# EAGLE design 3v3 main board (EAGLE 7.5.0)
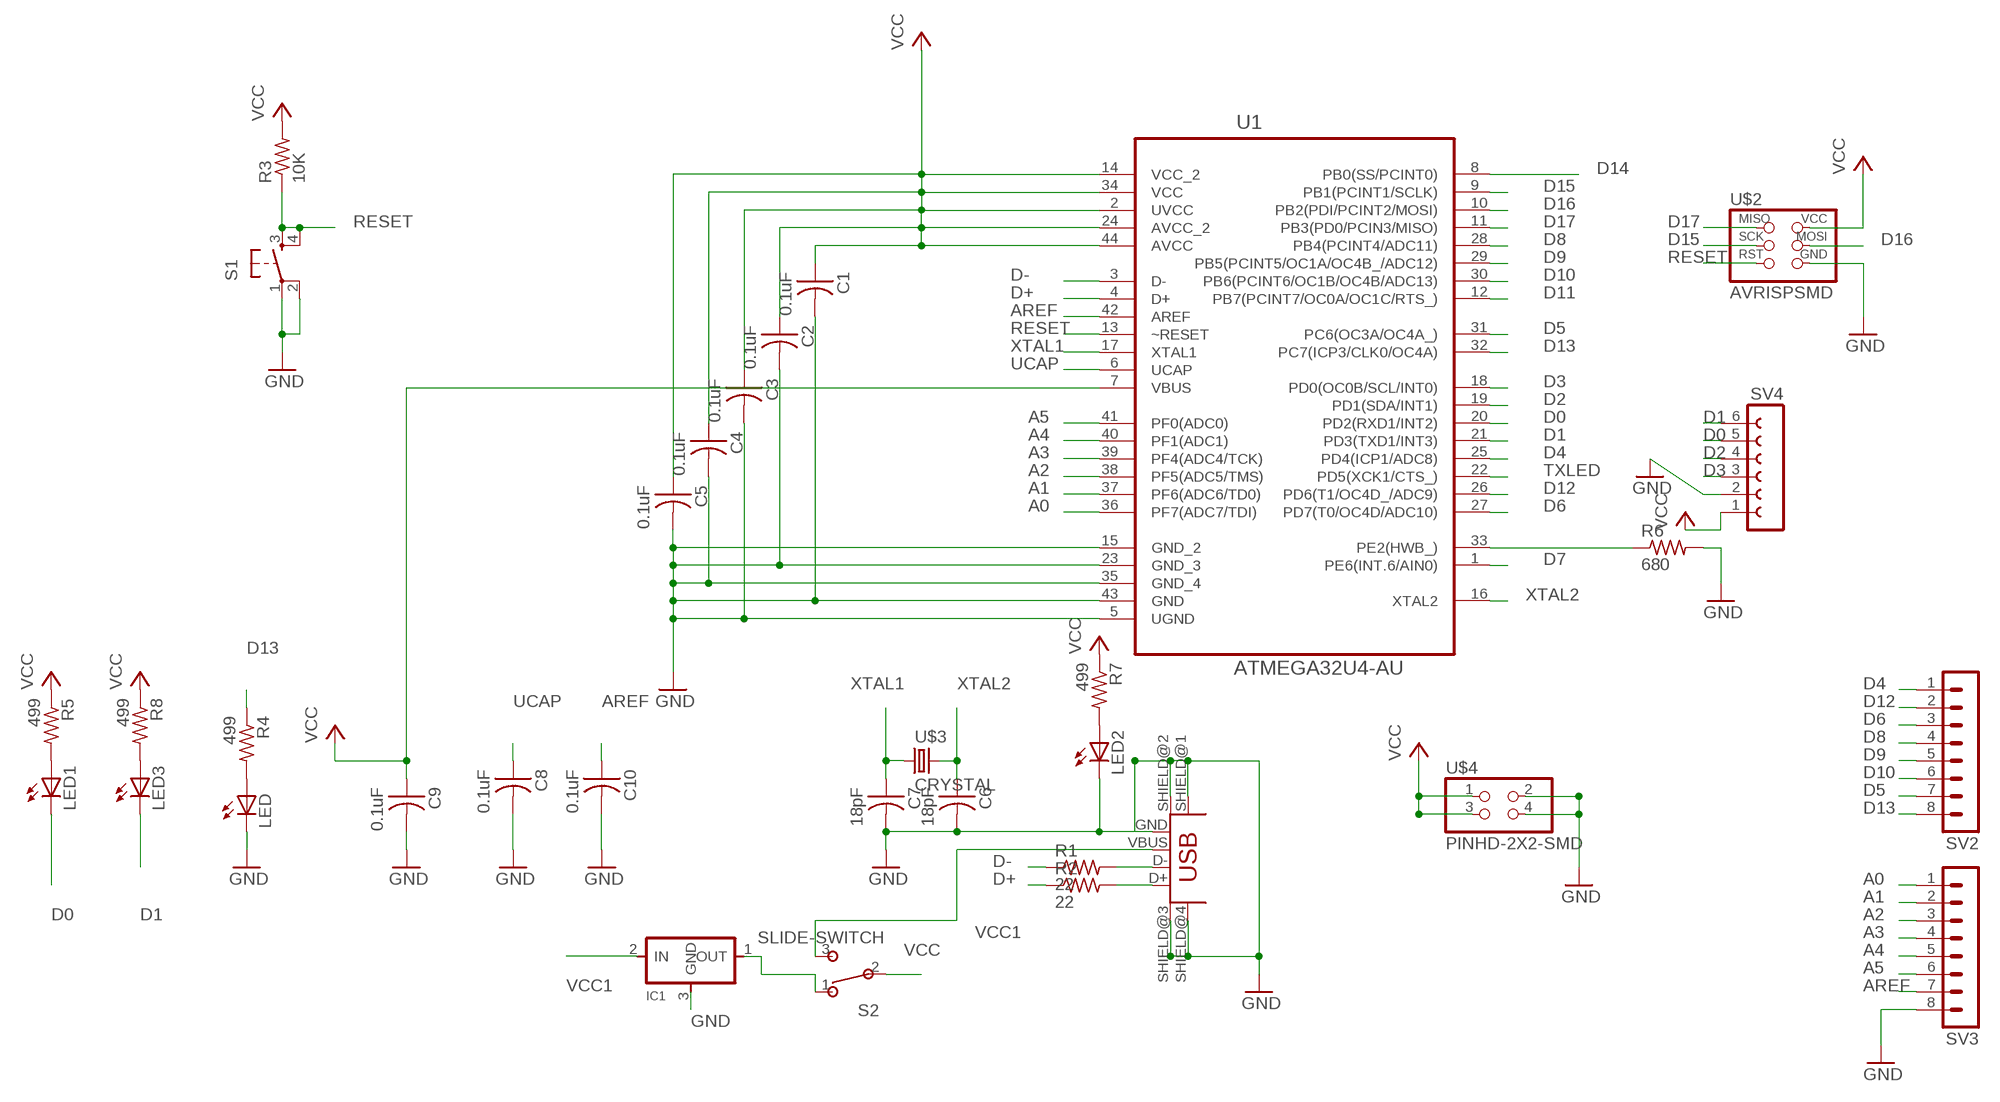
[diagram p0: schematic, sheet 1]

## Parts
C1  0.1uF  CAP-US1206FAB  [C1206FAB]
C2  0.1uF  CAP-US1206FAB  [C1206FAB]
C3  0.1uF  CAP-US1206FAB  [C1206FAB]
C4  0.1uF  CAP-US1206FAB  [C1206FAB]
C5  0.1uF  CAP-US1206FAB  [C1206FAB]
C6  18pF  CAP-US1206FAB  [C1206FAB]
C7  18pF  CAP-US1206FAB  [C1206FAB]
C8  0.1uF  CAP-US1206FAB  [C1206FAB]
C9  0.1uF  CAP-US1206FAB  [C1206FAB]
C10  0.1uF  CAP-US1206FAB  [C1206FAB]
IC1  REGULATORSOT23  [SOT23]
LED  LED1206  [1206]
LED1  LED1206  [1206]
LED2  LED1206  [1206]
LED3  LED1206  [1206]
R1  22  RES-US1206FAB  [R1206FAB]
R2  22  RES-US1206FAB  [R1206FAB]
R3  10K  RES-US1206FAB  [R1206FAB]
R4  499  RESISTOR1206  [1206]
R5  499  RESISTOR1206  [1206]
R6  680  RES-US1206FAB  [R1206FAB]
R7  499  RESISTOR1206  [1206]
R8  499  RESISTOR1206  [1206]
S1  6MM_SWITCH6MM_SWITCH  [6MM_SWITCH]
S2  SLIDE-SWITCH  [AYZ0102AGRLC]
SV2  MA08-1  [MA08-1]
SV3  MA08-1  [MA08-1]
SV4  FE06-1  [FE06]
U1  ATMEGA32U4-AU  [QFP80P1200X1200X120-44N]
U$1  USB_MINIB  [USB_MINIB]
U$2  AVRISPSMD  [2X03SMD]
U$3  CRYSTAL  [2-SMD-5X3MM]
U$4  PINHD-2X2-SMD  [2X02SMD]

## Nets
A0: SV3.1 U1.36(PF7(ADC7/TDI))
A1: SV3.2 U1.37(PF6(ADC6/TD0))
A2: SV3.3 U1.38(PF5(ADC5/TMS))
A3: SV3.4 U1.39(PF4(ADC4/TCK))
A4: SV3.5 U1.40(PF1(ADC1))
A5: SV3.6 U1.41(PF0(ADC0))
AREF: C10.1 SV3.7 U1.42(AREF)
D0: LED1.2(C) SV4.5 U1.20(PD2(RXD1/INT2))
D1: LED3.2(C) SV4.6 U1.21(PD3(TXD1/INT3))
D2: SV4.4 U1.19(PD1(SDA/INT1))
D3: SV4.3 U1.18(PD0(OC0B/SCL/INT0))
D4: SV2.1 U1.25(PD4(ICP1/ADC8))
D5: SV2.7 U1.31(PC6(OC3A/OC4A_))
D6: SV2.3 U1.27(PD7(T0/OC4D/ADC10))
D7: U1.1(PE6(INT.6/AIN0))
D8: SV2.4 U1.28(PB4(PCINT4/ADC11))
D9: SV2.5 U1.29(PB5(PCINT5/OC1A/OC4B_/ADC12))
D10: SV2.6 U1.30(PB6(PCINT6/OC1B/OC4B/ADC13))
D11: U1.12(PB7(PCINT7/OC0A/OC1C/RTS_))
D12: SV2.2 U1.26(PD6(T1/OC4D_/ADC9))
D13: R4.1 SV2.8 U1.32(PC7(ICP3/CLK0/OC4A))
D14: U1.8(PB0(SS/PCINT0))
D15: U1.9(PB1(PCINT1/SCLK)) U$2.3(SCK)
D16: U1.10(PB2(PDI/PCINT2/MOSI)) U$2.4(MOSI)
D17: U1.11(PB3(PD0/PCIN3/MISO)) U$2.1(MISO)
D+: R2.1 U1.4(D+)
D-: R1.1 U1.3(D-)
GND: C1.2 C2.2 C3.2 C4.2 C5.2 C6.2 C7.2 C8.2 C9.2 C10.2 IC1.3(GND) LED2.2(C) LED.2(C) R6.2 S1.1(P) S1.2(P1) SV3.8 SV4.2 U1.5(UGND) U1.15(GND_2) U1.23(GND_3) U1.35(GND_4) U1.43(GND) U$1.GND U$1.SHIELD@1(SHIELD) U$1.SHIELD@2(SHIELD1) U$1.SHIELD@3(SHIELD2) U$1.SHIELD@4(SHIELD3) U$2.6(GND) U$4.2 U$4.4
N$1: R1.2 U$1.D-
N$2: R2.2 U$1.D+
N$3: LED.1(A) R4.2
N$4: LED1.1(A) R5.2
N$5: LED2.1(A) R7.2
N$6: LED3.1(A) R8.2
N$10: IC1.1(OUT) S2.1
N$35: R6.1 U1.33(PE2(HWB_))
RESET: R3.1 S1.3(S) S1.4(S1) U1.13(~RESET) U$2.5(RST)
TXLED: U1.22(PD5(XCK1/CTS_))
UCAP: C8.1 U1.6(UCAP)
VCC: C1.1 C2.1 C3.1 C4.1 C5.1 C9.1 R3.2 R5.1 R7.1 R8.1 S2.2 SV4.1 U1.2(UVCC) U1.7(VBUS) U1.14(VCC_2) U1.24(AVCC_2) U1.34(VCC) U1.44(AVCC) U$2.2(VCC) U$4.1 U$4.3
VCC1: IC1.2(IN) S2.3 U$1.VBUS
XTAL1: C7.1 U1.17(XTAL1) U$3.P$1
XTAL2: C6.1 U1.16(XTAL2) U$3.P$2

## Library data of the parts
C1-C10 = fab:CAP-US
IC1 = fab:REGULATOR
LED LED1-LED3 = ng:LED
R1-R3 R6 = fab:RES-US: Resistor (US Symbol)
R4 R5 R7 R8 = ng:RESISTOR
S1 = ng:6MM_SWITCH: OMRON SWITCH
S2 = fab:SLIDE-SWITCH: SMD slide-switch AYZ0102AGRLC as found in the fablab inventory. Includes the mounting holes. Made by Zaerc.
SV2 SV3 = con-lstb:MA08-1: PIN HEADER; OC_FARNELL: unknown; OC_NEWARK: unknown
SV4 = con-lsta:FE06-1: FEMALE HEADER; OC_FARNELL: unknown; OC_NEWARK: unknown
U1 = Atmel_By_element14_Batch_1:ATMEGA32U4-AU: 8-bit Microcontroller with ISP Flash and USB Controller; MPN: ATMEGA32U4-AU; OC_FARNELL: 1748525; OC_NEWARK: 26R5633; PACKAGE: TQFP-44; SUPPLIER: Atmel
U$1 = fab:USB_MINIB
U$2 = fab:AVRISP
U$3 = fab:CRYSTAL
U$4 = fab:PINHD-2X2-SMD

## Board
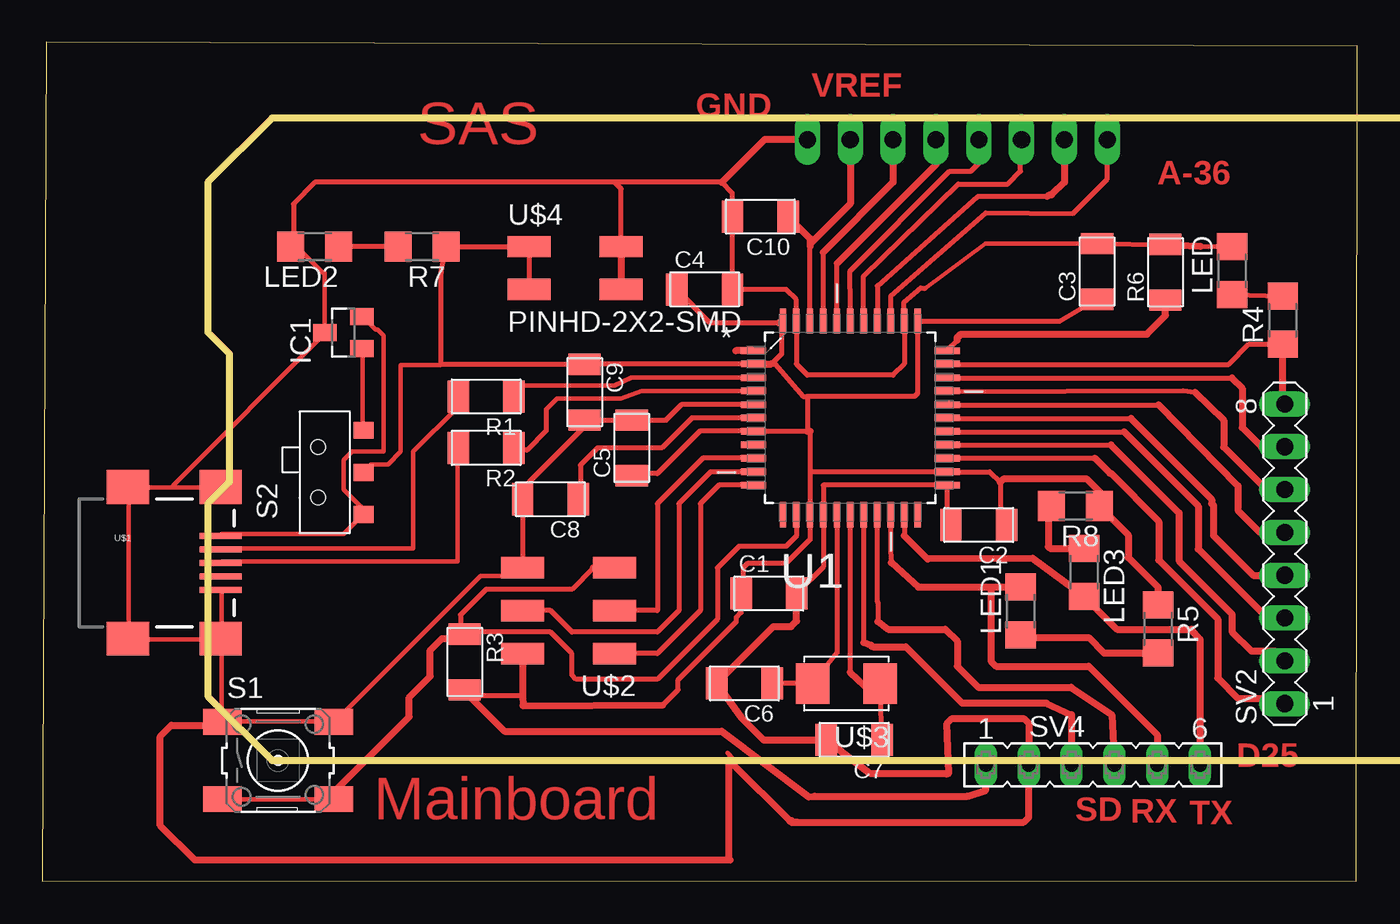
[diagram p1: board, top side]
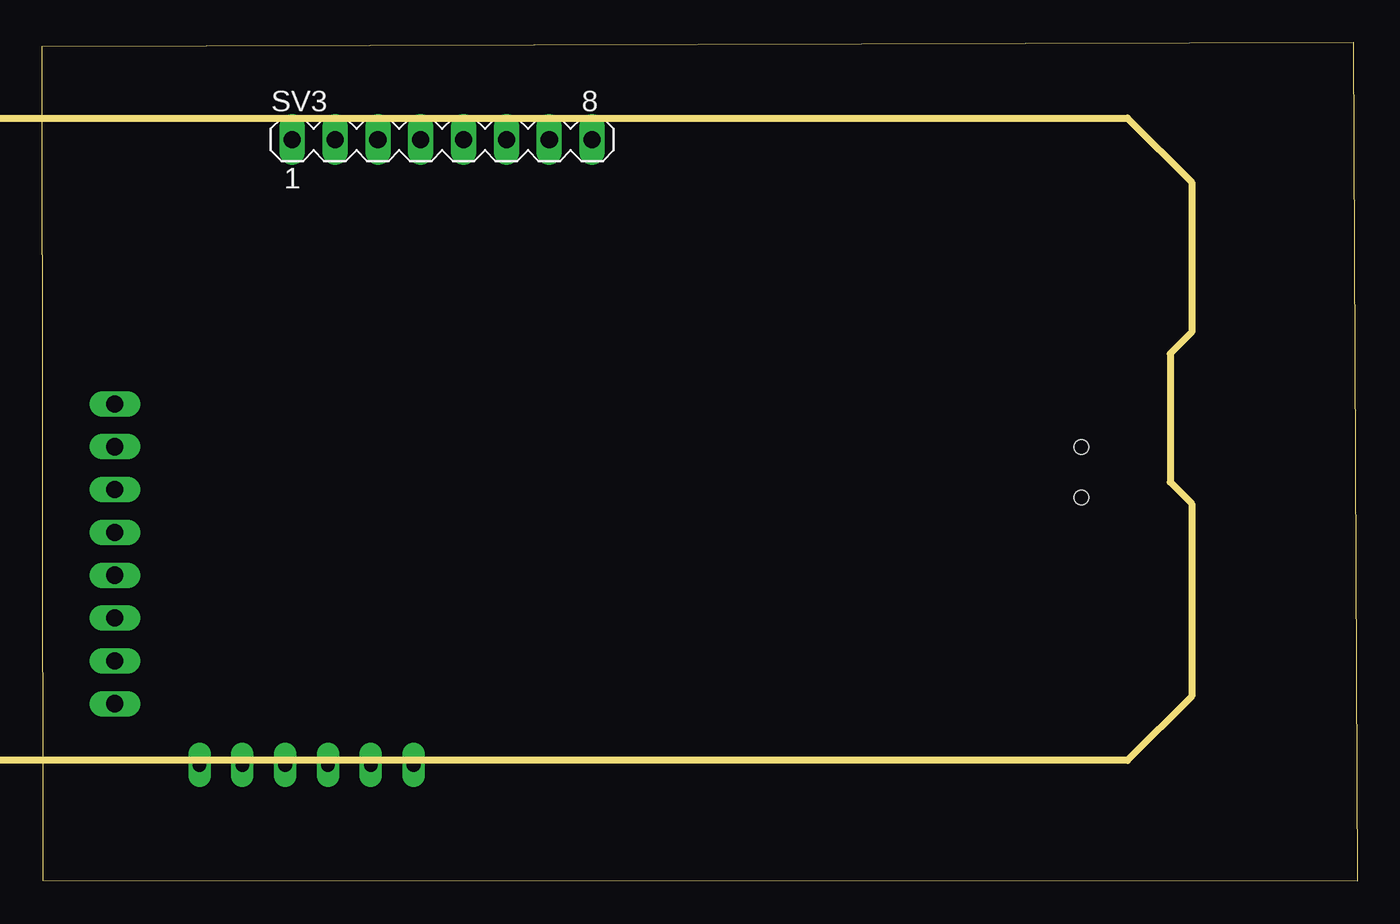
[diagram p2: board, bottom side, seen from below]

Size 77.99 x 49.78 mm. Coordinates in mm from the lower left corner, seen from the top.
Outline: 0,0 77.94,0.05 77.99,49.53 0.25,49.78 0,0
Copper layers (1*16): Top 0.035mm / dielectric 1.5mm / Bottom 0.035mm
Design rules "default *": minimum track width 10mil, minimum drill 24mil, track to track 0.4mm, track to pad 0.4mm, pad to pad 0.4mm, via to via 0.4mm, smd to smd 0.4mm, copper to edge 40mil, drill to drill 0.4mm, minimum pad ring 10mil, minimum via ring 8mil, stop-mask expansion 4mil, vias tented up to drill 0mil, thermal gap 10mil
Milling: area 9.8,7.2 to 110.2,45.3

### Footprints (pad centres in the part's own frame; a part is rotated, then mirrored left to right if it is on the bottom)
C1206FAB = smd 1.27 x 1.905: 1 -1.651,0; 2 1.651,0
SOT23 = smd 1 x 1.4: 1 -0.95,-1.1; 2 0.95,-1.1; 3 0,1.1
1206 = smd 1.6 x 1.803: 1 -1.422,0; 2 1.422,0
R1206FAB = smd 1.27 x 1.905: 1 -1.651,0; 2 1.651,0
6MM_SWITCH = smd 2.286 x 1.524: 1 -3.302,2.286; 2 3.302,2.286; 3 -3.302,-2.286; 4 3.302,-2.286
AYZ0102AGRLC = smd 1 x 1.2: 1 2.5,-2.3; 2 0,-2.3; 3 -2.5,-2.3 | hole 0.85: -1.5,0.4; 1.5,0.4
MA08-1 = drill 1.016 long: 1 -8.89,0; 2 -6.35,0; 3 -3.81,0; 4 -1.27,0; 5 1.27,0; 6 3.81,0; 7 6.35,0; 8 8.89,0
FE06 = drill 0.813 long: 1 -6.35,0; 2 -3.81,0; 3 -1.27,0; 4 1.27,0; 5 3.81,0; 6 6.35,0
QFP80P1200X1200X120-44N = smd 1.5 x 0.38: 1 -5.74,3.988; 2 -5.74,3.2; 3 -5.74,2.388; 4 -5.74,1.6; 5 -5.74,0.787; 6 -5.74,0; 7 -5.74,-0.787; 8 -5.74,-1.6; 9 -5.74,-2.388; 10 -5.74,-3.2; 11 -5.74,-3.988; 23 5.74,-3.988; 24 5.74,-3.2; 25 5.74,-2.388; 26 5.74,-1.6; 27 5.74,-0.787; 28 5.74,0; 29 5.74,0.787; 30 5.74,1.6; 31 5.74,2.388; 32 5.74,3.2; 33 5.74,3.988 | smd 0.38 x 1.5: 12 -3.988,-5.74; 13 -3.2,-5.74; 14 -2.388,-5.74; 15 -1.6,-5.74; 16 -0.787,-5.74; 17 0,-5.74; 18 0.787,-5.74; 19 1.6,-5.74; 20 2.388,-5.74; 21 3.2,-5.74; 22 3.988,-5.74; 34 3.988,5.74; 35 3.2,5.74; 36 2.388,5.74; 37 1.6,5.74; 38 0.787,5.74; 39 0,5.74; 40 -0.787,5.74; 41 -1.6,5.74; 42 -2.388,5.74; 43 -3.2,5.74; 44 -3.988,5.74
USB_MINIB = smd 2.5 x 0.35: D+ 3.77,0; D- 3.77,0.8; GND 3.77,-1.6; ID 3.77,-0.8; VBUS 3.77,1.6 | smd 2.5 x 2: SHIELD@1 -1.73,-4.5; SHIELD@2 -1.73,4.5; SHIELD@3 3.77,4.5; SHIELD@4 3.77,-4.5
2X03SMD = smd 2.54 x 1.27: 1 -2.54,2.54; 2 2.92,2.54; 3 -2.54,0; 4 2.92,0; 5 -2.54,-2.54; 6 2.92,-2.54
2-SMD-5X3MM = smd 2 x 2.4: P$1 -2,0; P$2 2,0
2X02SMD = smd 2.54 x 1.27: 1 -2.54,1.27; 2 2.92,1.27; 3 -2.54,-1.27; 4 2.92,-1.27

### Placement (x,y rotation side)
C1  43.09,17.08 0 top
C2  55.54,21.14 180 top
C3  62.56,36.18 90 top
C4  39.28,35.11 0 top
C5  34.97,25.71 90 top
C6  41.64,11.74 180 top
C7  48.15,8.39 180 top
C8  30.14,22.66 180 top
C9  32.17,29.01 270 top
C10  42.59,39.43 180 top
IC1  17.86,32.56 90 top
LED  70.57,36.23 90 top
LED1  58.03,16.04 90 top
LED2  16.17,37.65 180 top
LED3  61.78,18.33 270 top
R1  26.33,28.76 180 top
R2  26.33,25.71 180 top
R3  25.06,13.01 270 top
R4  73.57,33.28 90 top
R5  66.17,14.97 270 top
R6  66.61,36.13 90 top
R7  22.52,37.65 180 top
R8  61.27,22.27 180 top
S1  13.99,7.17 0 top
S2  16.76,24.26 90 top
SV2  73.68,19.43 90 top
SV3  54.27,44 0 bottom
SV4  62.31,6.91 0 top
U1  47.92,27.49 0 top
U$1  6.82,18.89 0 top
U$2  31.41,16.06 180 top
U$3  47.69,11.74 180 top
U$4  31.41,36.38 0 top

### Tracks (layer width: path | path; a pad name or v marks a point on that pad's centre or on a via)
A0
  Top 0.305: SV3.1 63.16,41.66 61.11,39.61 55.96,39.66 50.31,34.71 U1.36
A1
  Top 0.305: 59.6,40.64 55.49,40.64 49.52,35.32 U1.37
  Top 0.406: SV3.2 60.62,41.46 59.85,40.73 59.6,40.64
A2
  Top 0.305: U1.38 48.71,35.91 54.31,41.36 57.26,41.36 58.01,42.11 58.01,43.21 58.06,43.26 58.06,43.16 58.08,43.18 SV3.3
A3
  Top 0.254: 55.59,43.98 55.63,43.98 SV3.4
  Top 0.305: U1.39 47.92,33.85 47.91,33.86 47.91,35.1 47.92,35.11 47.91,35.12 47.91,36.21 53.81,42.11 55.06,42.11 55.54,42.59 55.54,43.26
  Top 0.406: 55.54,42.73 55.54,43.26 SV3.4 | 55.59,43.56 55.59,43.98 55.59,44.3
A4
  Top 0.305: U1.40 47.13,36.64
  Top 0.406: SV3.5 53,42.51 47.13,36.64
A5
  Top 0.305: U1.41 46.32,37.32
  Top 0.406: SV3.6 50.46,41.46 46.32,37.32
AREF
  Top 0.305: U1.42 45.53,37.65
  Top 0.406: C10.1 45.53,38.13 45.53,37.8 | SV3.7 47.92,40.19 45.53,37.8 | 45.53,37.8 45.53,37.65
D0
  Top 0.305: U1.20 50.31,19.56 50.36,18.91
  Top 0.406: 50.36,18.91 51.96,17.46 56.26,17.46 | 56.26,17.46 LED1.2 | 56.26,17.46 56.26,13.06 56.56,12.76 62.06,12.76 66.12,8.7 SV4.5
D1
  Top 0.305: U1.21 51.12,20.5
  Top 0.406: SV4.6 68.66,14.36 68.16,14.96 63.73,14.96 LED3.2 58.73,19.16 52.51,19.11 51.12,20.5
D2
  Top 0.254: 49.51,21.51 49.51,21.73 U1.19
  Top 0.305: 49.56,21.56 49.51,21.51 49.51,16.61 49.56,16.56 49.56,15.41
  Top 0.406: 49.56,15.41 50.16,14.96 53.56,14.96 54.26,14.26 54.26,12.76 55.51,11.51 61.01,11.51 63.43,9.89 SV4.4
D3
  Top 0.305: U1.18 48.71,14.16
  Top 0.406: 48.71,14.16 49.16,14.01 49.26,13.91 51.21,13.91 54.56,10.56 59.56,10.56 61.04,9.88 SV4.3
D4
  Top 0.305: U1.25 62.42,25.1
  Top 0.406: 62.42,25.1 63.31,24.21 63.36,24.21 66.21,21.36 66.21,19.06 69.71,15.56 69.71,12.06 70.91,10.86 73.36,10.86 SV2.1
D5
  Top 0.254: 53.76,29.86 U1.31
  Top 0.305: 53.68,29.86 53.76,29.86 70.56,29.86
  Top 0.406: 70.56,29.86 71.16,29.26 71.16,26.91 72.29,25.78 SV2.7
D6
  Top 0.254: U1.27 53.76,26.73 53.76,26.66
  Top 0.305: 53.7,26.66 53.76,26.66 64.16,26.66
  Top 0.406: 64.16,26.66 68.56,22.26 68.56,19.71 72.65,15.62 SV2.3
D7
  Top 0.406: U1.1 41.14,31.48
D8
  Top 0.254: U1.28 53.76,27.48 53.76,27.46
  Top 0.305: 53.69,27.51 53.74,27.46 53.76,27.46 64.56,27.46
  Top 0.406: 64.56,27.46 69.36,22.66 69.36,22.41 69.46,22.31 69.46,20.51 71.81,18.16 SV2.4
D9
  Top 0.254: U1.29 53.76,28.36 53.76,28.26
  Top 0.305: 53.73,28.26 53.76,28.26 66.21,28.26
  Top 0.406: 66.21,28.26 70.91,23.46 70.91,22.01 72.22,20.7 SV2.5
D10
  Top 0.254: U1.30 53.76,29.11 53.76,29.06
  Top 0.305: 53.74,29.06 53.76,29.06 67.66,29.11 68.36,29.01
  Top 0.406: 72.33,23.24 SV2.6 72.58,23.24 70.06,25.76 70.06,27.36 68.36,29.01
D12
  Top 0.305: U1.26 63.38,25.89
  Top 0.406: 63.38,25.89 67.41,21.86 67.41,19.01 70.56,15.86 70.56,14.81 71.71,13.66 73.1,13.66 SV2.2
D13
  Top 0.305: U1.32 53.69,30.66 70.36,30.66 71.56,31.86 R4.1
  Top 0.406: SV2.8 73.57,28.43 R4.1
D15
  Top 0.305: U1.9 39.18,25.1 36.49,22.41 36.49,16.06 U$2.3
D16
  Top 0.305: U1.10 39.64,24.29 37.76,22.41 37.76,16.06 36.49,14.79 31.41,14.79 30.14,16.06 U$2.4
D17
  Top 0.305: U1.11 40.12,23.5 39.03,22.41 39.03,16.06 36.49,13.52 U$2.1
D+
  Top 0.254: U1.4 35.55,29.09 34.33,28.63 30.52,28.63 29.89,28
  Top 0.305: 29.89,28 29.89,26.73 28.74,25.59 28.11,25.59 R2.1
D-
  Top 0.254: U1.3 34.94,29.88 33.95,29.39 28.11,29.39
  Top 0.305: 28.11,29.39 27.85,28.89 R1.1
GND
  Top 0.254: 52.36,35.16 55.93,37.83 C3.2 | U$1.SHIELD@4 10.63,14.36 10.63,9.48 S1.1 10.76,9.48 11.21,9.48 17.26,9.48 S1.2 | U$1.SHIELD@4 10.51,14.36 5.13,14.36 U$1.SHIELD@1 5.13,14.48 5.13,23.23 U$1.SHIELD@2 5.13,23.36 7.76,23.36 | U$1.GND 10.63,17.23 10.63,14.48 U$1.SHIELD@4 | LED2.2 15.01,37.73 16.63,36.11 16.76,36.11 IC1.3 16.76,32.48 7.76,23.48 7.76,23.36 | 7.76,23.36 10.51,23.36 U$1.SHIELD@3 | U$2.6 28.38,18.48 28.01,18.11 26.01,18.11 17.38,9.48 S1.2 | 40.63,7.61 41.01,7.23 41.01,7.11 40.91,7.01 | 17.38,9.36 S1.2
  Top 0.305: U1.5 37.91,28.28 37,27.36 C5.2 C9.2 | C3.2 R6.2 | 68.7,37.67 LED.2 | 53.66,21.37 U1.23 46.32,23.5 U1.15 46.32,18.65 C1.2 | C8.2 U$2.6 | 33.95,41.46 40.3,41.46 40.93,40.83 C10.2 C4.2 44.11,35.11 44.72,34.5 U1.43 44.72,30.69 45.38,30.03 50.46,30.03 51.12,30.69 U1.35 51.11,33.24 51.11,34.36 52.11,35.21 52.36,35.16 | 33.95,41.46 16.17,41.46 14.9,40.19 14.9,37.8 | U$4.4 34.33,41.08 33.95,41.46 | 32.17,26.98 28.87,23.68 28.87,23.04
  Top 0.406: R6.2 68.7,37.67 | 53.66,21.37 C2.2 | U$4.2 U$4.4 | C9.2 32.17,26.98 | 28.87,23.04 C8.2 | U$2.6 | 44.74,16.7 C1.2 44.74,15.45 44.41,15.11 43.36,15.11 C6.2 41.44,9.73 42.78,8.39 C7.2 49.08,6.41 53.76,6.41 | 14.9,37.8 LED2.2 | SV3.8 42.84,44 40.3,41.46 | 53.76,6.41 53.61,6.36 | 53.76,6.41 53.66,9.36 53.96,9.66 58.21,9.66 58.5,9.37 58.5,7.41 | 58.51,7.92 58.5,7.41 | 58.5,7.41 SV4.2 58.5,3.8 58.21,3.51 44.41,3.51 44.31,3.61 | 44.31,3.61 44.46,3.61 44.46,3.51 44.76,3.51 | 44.31,3.61 40.91,7.01 40.71,7.21 40.71,1.36 40.81,1.26 9.06,1.26 7.01,3.31 7.01,8.61 7.66,9.26 10.98,9.26 11.21,9.48
N$1
  Top 0.254: R1.2 24.63,28.11 22.01,25.48 22.01,19.73 10.63,19.73 U$1.D-
  Top 0.406: 24.68,28.29 R1.2 24.68,28.46
N$2
  Top 0.254: R2.2 24.63,25.61 24.63,18.98 10.63,18.98 U$1.D+
N$3
  Top 0.305: LED.1 R4.2
N$4
  Top 0.406: LED1.1 58.19,14.46 62.06,14.46 62.97,13.55 R5.2
N$5
  Top 0.305: R7.2 LED2.1
N$6
  Top 0.406: R8.2 59.66,22.08 59.66,19.86 59.76,19.76 LED3.1
N$10
  Top 0.254: S2.1 19.01,26.86 19.01,31.61 IC1.1
N$35
  Top 0.305: 54.26,32.08 U1.33
  Top 0.406: 54.26,32.08 54.26,32.26 54.46,32.46 65.51,32.46 66.61,33.56 R6.1
RESET
  Top 0.254: S1.3 10.76,4.86 17.26,4.86 S1.4
  Top 0.305: U1.13 44.72,20.48 44.11,19.87 41.32,19.87 40.05,18.6 40.05,15.55 36.49,12 31.66,12 31.41,12.25 31.41,13.52 30.14,14.79 25.19,14.79 | 32.68,18.6 31.41,17.33 26.33,17.33 24.81,15.81 24.81,14.92 R3.1
  Top 0.406: 25.19,14.79 R3.1 24.81,14.41 23.71,14.41 23.01,13.71 23.01,12.16 21.76,10.91 21.76,9.76 17.29,5.29 S1.4 | U$2.5 32.68,18.6
UCAP
  Top 0.305: U1.6 38.52,27.49 36.74,25.71 32.93,25.71 31.92,24.7 31.92,22.79 C8.1
VCC
  Top 0.254: S2.2 19.13,24.36 19.51,24.73 20.51,24.73 21.26,25.48 21.26,30.61 23.63,30.61 23.66,30.66
  Top 0.305: 43.25,30.69 43.86,31.3 43.86,33.15 | 32.2,30.69 U1.2 43.45,30.69 45.13,28.76 45.38,28.76 | C9.1 23.66,30.66 23.66,36.1 R7.1 U$4.1 U$4.3 | C3.1 60.34,33.23 U1.34 51.91,28.94 51.73,28.76 45.38,28.76 | 56.81,21.52 56.81,23.68 56.2,24.29 U1.24 45.53,24.29 | 43.68,33.13 39.61,33.13 C4.1 | 41.57,17.2 41.57,18.6 41.82,18.85 44.11,18.85 45.53,20.28 U1.14 45.53,24.29 | 45.53,26.7 45.53,24.29 | 45.38,28.76 45.38,26.7 U1.7 39,26.7 36.49,24.19 34.59,24.19 C5.1 | R3.2 25.4,11.02 28.5,11.02 | 36.81,10.46 37.71,11.36 37.71,11.96 41.16,15.41 41.16,15.66 41.44,15.94 C1.1
  Top 0.406: U1.2 43.25,30.69 | 43.86,33.15 U1.44 43.68,33.13 | 51.98,33.15 U1.34 | 32.2,30.69 C9.1 | 37.76,34.98 C4.1 | 56.81,21.52 C2.1 | 41.57,17.2 C1.1 41.51,17.01 | 45.38,26.7 45.53,26.7 | 56.81,23.68 56.99,23.86 61.96,23.86 62.74,23.08 R8.1 64.41,20.55 64.41,19.21 66.17,17.45 R5.1 | 56.01,7.86 SV4.1 55.96,5.41 54.86,5.06 45.81,5.06 45.46,5.01 40.31,8.91 27.41,8.91 25.01,11.31 R3.2 | 36.81,10.46 28.51,10.41 28.5,11.02 28.49,11.58 U$2.2
VCC1
  Top 0.254: U$1.VBUS 10.63,20.61 17.88,20.61 19.01,21.73 S2.3 19.01,21.86 19.01,22.11 17.88,23.23 17.88,24.98 18.38,25.48 20.26,25.48 20.26,32.36 19.88,32.73 19.76,32.73 19.01,33.48 IC1.2
XTAL1
  Top 0.254: U1.17 47.88,21.73 47.91,21.71
  Top 0.305: C7.1 49.71,11.23 U$3.P$1 | 47.91,21.71 47.91,12.41
  Top 0.406: 47.91,12.41 49.14,11.23 49.71,11.23
XTAL2
  Top 0.305: C6.1 U$3.P$2 47.13,13.58 U1.16

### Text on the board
Top: VREF | GND | SAS | A-36 | D25 | Mainboard | SD | RX | TX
